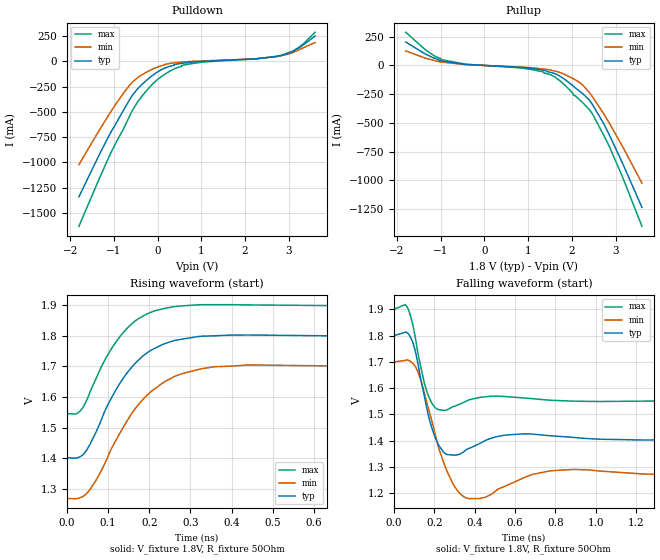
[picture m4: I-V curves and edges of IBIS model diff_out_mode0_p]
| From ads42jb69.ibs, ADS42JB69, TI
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|   diff_out_mode0 Model
[Model]   diff_out_mode0_p
Model_type   Output
Polarity   Non-Inverting
Vmeas = 1.611
Vref = 1.8
Cref = 0.5pF
Rref = 50
|   typ   min   max
|   (nom PVT)   (fast PVT)   (slow PVT)
C_comp   2.771e-12   2.341e-12   2.803e-12
[Model spec]
|subparameter   typ   min   max
Vmeas   1.611   1.505   1.7254
| Where nom  PVT is Nominal Process, 1.8V, 25C
|   Fast PVT is Strong Process,  1.9V, -40C
|   Slow PVT is Weak Process,   1.7V, 125C
[Voltage Range]   1.8   1.7   1.9
|Junction Temperature
[Temperature Range]   25   125   -40
[Pullup Reference]   1.8   1.7   1.9
[Pulldown Reference]   0   0   0
[Power Clamp Reference]   1.8   1.7   1.9
[GND Clamp Reference]   0   0   0
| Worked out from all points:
|   slope of the pulldown table from 0 to 0.27 V, typ, clamps not added: 5.02 ohm
|   slope of the pullup table from 0 to 0.27 V, typ, clamps not added: 49.4 ohm
|   falling waveform, V_fixture 1.8V, R_fixture 50Ohm: 20-80 % time 63.6ps typ, 89.7ps min, 54.2ps max; typ from 1.8 V to 1.4 V
|   rising waveform, V_fixture 1.8V, R_fixture 50Ohm: 20-80 % time 103ps typ, 118ps min, 92.7ps max; typ from 1.4 V to 1.8 V
[Pulldown]
|   Voltage   I(typ)   I(min)   I(max)
-1.8V     -1.34A     -1.022A    -1.632A
-1.078V   -708.2mA   -503.6mA   -912.9mA
-617.4mV  -362.5mA   -224.1mA   -519.7mA
-373.1mV  -234.5mA   -136.6mA   -352.8mA
-2.6mV    -104.5mA   -56.41mA   -179.8mA
381.6mV   -31.66mA   -14.11mA   -73.7mA
621mV     -15.45mA   -4.391mA   -34.61mA
1.082V    1.461mA    5.463mA    -5.442mA
2.252V    25.55mA    26.17mA    25.09mA
2.836V    58.76mA    57.27mA    60.53mA
3.247V    137.8mA    117.4mA    144.6mA
3.6V      250.8mA    186.5mA    287.9mA
[Pullup]
|   Voltage   I(typ)   I(min)   I(max)
-1.8V     203.7mA    126.2mA    288.4mA
-1.342V   97.45mA    62.7mA     134.5mA
-1.004V   40.03mA    30.51mA    51.97mA
-450mV    9.478mA    7.89mA     12.08mA
1.082V    -26.41mA   -20.41mA   -36.04mA
1.357V    -42.28mA   -31.39mA   -57.53mA
1.695V    -86.58mA   -57.19mA   -124.8mA
2.154V    -218.3mA   -143.2mA   -291.1mA
2.477V    -345.3mA   -277mA     -427.9mA
2.853V    -603.1mA   -500.6mA   -702.9mA
3.176V    -867.5mA   -718.8mA   -989.4mA
3.6V      -1.235A    -1.023A    -1.399A
[Ramp]
R_load = 50
|   typ   min   max
dV/dt_r   0.104408/5.88701e-11   0.13755/7.39903e-11  0.0846468/4.82495e-11
dV/dt_f   0.237884/6.34098e-11   0.258233/8.94316e-11   0.210173/5.41391e-11
[Falling Waveform]
V_fixture = 1.8V
V_fixture_min = 1.7V
V_fixture_max = 1.9V
R_fixture = 50Ohm
|   Time   V(typ)   V(min)   V(max)
0s        1.799V     1.699V     1.899V
60ps      1.813V     1.706V     1.915V
92ps      1.777V     1.695V     1.845V
152ps     1.565V     1.576V     1.615V
200ps     1.421V     1.438V     1.529V
290ps     1.345V     1.24V      1.528V
360ps     1.367V     1.181V     1.551V
552ps     1.421V     1.227V     1.568V
782ps     1.418V     1.286V     1.554V
2.198ns   1.403V     1.269V     1.549V
[Rising Waveform]
V_fixture = 1.8V
V_fixture_min = 1.7V
V_fixture_max = 1.9V
R_fixture = 50Ohm
|   Time   V(typ)   V(min)   V(max)
0s        1.402V     1.269V     1.546V
32ps      1.405V     1.271V     1.555V
56ps      1.446V     1.298V     1.618V
106ps     1.592V     1.427V     1.754V
162ps     1.705V     1.555V     1.845V
196ps     1.746V     1.608V     1.873V
238ps     1.775V     1.651V     1.89V
330ps     1.799V     1.693V     1.902V
444ps     1.803V     1.705V     1.901V
2.108ns   1.798V     1.698V     1.899V
